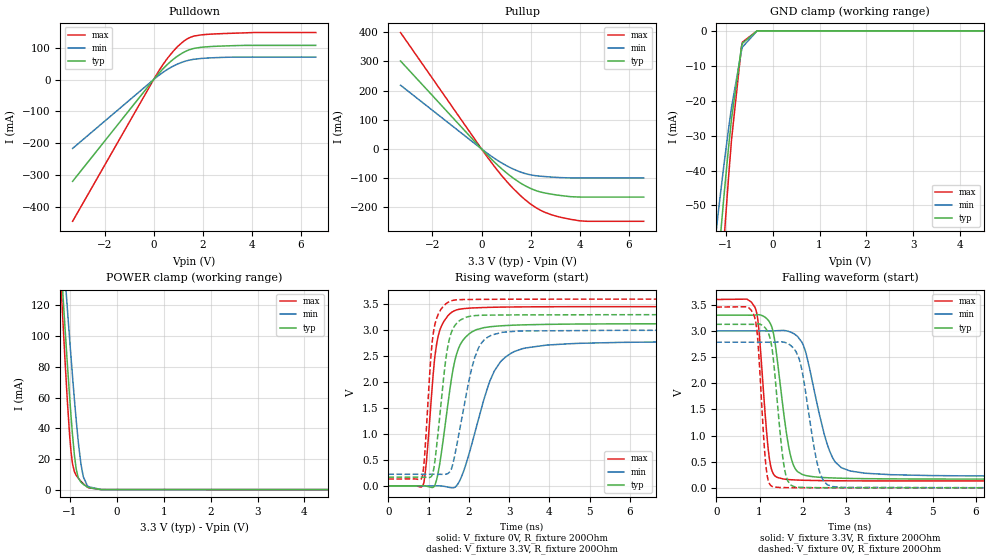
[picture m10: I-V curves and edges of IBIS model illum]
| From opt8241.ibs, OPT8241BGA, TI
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|   illum Model
[Model]   illum
Model_type   I/O
Polarity   Non-Inverting
Enable   Active-High
Vinl = 0.99
Vinh = 2.31
Vmeas = 1.65
Vref = 0
Cref = 2pF
Rref = 200
|   typ   min   max
|   (nom PVT)   (fast PVT)   (slow PVT)
C_comp   2.708e-12   2.507e-12   2.914e-12
[Model spec]
|subparameter
Vinl   0.99   0.90   1.08
Vinh   2.31   2.10   2.52
| Where nom  PVT is Nominal Process, 3.3V, 27C
|   Fast PVT is Strong Process,  3.6V, -40C
|   Slow PVT is Weak Process,   3V, 125C
[Voltage Range]   3.3   3   3.6
|Junction Temperature
[Temperature Range]   27   125   -40
[Pullup Reference]   3.3   3   3.6
[Pulldown Reference]   0   0   0
[Power Clamp Reference]   3.3   3   3.6
[GND Clamp Reference]   0   0   0
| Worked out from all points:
|   slope of the pulldown table from 0 to 0.495 V, typ, clamps not added: 11.6 ohm
|   slope of the pullup table from 0 to 0.495 V, typ, clamps not added: 11.6 ohm
|   falling waveform, V_fixture 3.3V, R_fixture 200Ohm: 20-80 % time 297ps typ, 477ps min, 193ps max; typ from 3.3 V to 0.167 V
|   rising waveform, V_fixture 0V, R_fixture 200Ohm: 20-80 % time 365ps typ, 661ps min, 236ps max; typ from 0 V to 3.13 V
|   rising waveform, V_fixture 3.3V, R_fixture 200Ohm: 20-80 % time 271ps typ, 436ps min, 189ps max; typ from 0.168 V to 3.3 V
|   falling waveform, V_fixture 0V, R_fixture 200Ohm: 20-80 % time 217ps typ, 327ps min, 154ps max; typ from 3.12 V to 0 V
[Pulldown]
|   Voltage   I(typ)   I(min)   I(max)
-3.3V     -319.9mA   -216.5mA   -445.5mA
189mV     17.58mA    11.85mA    24.51mA
462mV     40.27mA    27mA       56.22mA
775.2mV   62.22mA    41.4mA     87.06mA
1.056V    78.05mA    51.51mA    109.5mA
1.251V    86.82mA    56.93mA    122mA
1.596V    97.13mA    63.25mA    135.8mA
2.165V    103mA      67.59mA    142mA
4.032V    107.5mA    70.78mA    147.8mA
6.6V      107.5mA    70.78mA    147.8mA
[GND Clamp]
|   Voltage   I(typ)   I(min)   I(max)
-3.3V     -1.553A    -1.315A    -1.789A
-1.214V   -75.2mA    -58.77mA   -96.04mA
-1.133V   -62.06mA   -49.14mA   -79.22mA
-1.033V   -46.78mA   -37.93mA   -59.46mA
-940.5mV  -33.68mA   -28.26mA   -42.33mA
-876mV    -25.29mA   -22mA      -31.29mA
-663mV    -4.673mA   -5.695mA   -4.527mA
-643.2mV  -3.575mA   -4.674mA   -3.252mA
-330mV    -4.518uA   -17.28uA   -5.664uA
6.6V      0A         0A         0A
[Pullup]
|   Voltage   I(typ)   I(min)   I(max)
-3.3V     301mA      218.2mA    398.3mA
1.2mV     -109.4uA   -79.25uA   -144.7uA
459mV     -39.81mA   -28.44mA   -53.04mA
855mV     -70.54mA   -49.65mA   -94.7mA
1.251V    -97.42mA   -67.29mA   -132mA
1.899V    -131.4mA   -86.9mA    -182.2mA
2.237V    -143.2mA   -91.82mA   -202mA
2.565V    -150.5mA   -94.39mA   -216.4mA
3.032V    -157.2mA   -97.16mA   -229.8mA
3.633V    -163.4mA   -99.07mA   -241mA
4.3V      -164.7mA   -99.07mA   -247.6mA
6.6V      -164.7mA   -99.07mA   -247.6mA
[POWER Clamp]
|   Voltage   I(typ)   I(min)   I(max)
-3.3V     1.269A     1.142A     1.492A
-1.219V   162.5mA    188.8mA    152mA
-1.14V    123.4mA    154.7mA    105.4mA
-1.099V   103.6mA    137.2mA    82.23mA
-1.065V   87.65mA    123mA      64.08mA
-974.4mV  47.89mA    86.2mA     24.75mA
-942mV    35.41mA    73.59mA    16.71mA
-864.6mV  13.5mA     45.43mA    9.371mA
-762mV    4.836mA    16.42mA    5.377mA
-714mV    3.486mA    8.521mA    3.853mA
-600mV    1.284mA    1.875mA    1.166mA
6.6V      0A         0A         0A
[Ramp]
R_load = 200
|   typ   min   max
dV/dt_r   1.87524/3.65085e-10   1.66989/6.58259e-10   2.07288/2.34928e-10
dV/dt_f   1.87941/2.96485e-10   1.66601/4.73757e-10   2.08068/1.93019e-10
[Falling Waveform]
V_fixture = 3.3V
V_fixture_min = 3V
V_fixture_max = 3.6V
R_fixture = 200Ohm
|   Time   V(typ)   V(min)   V(max)
0s        3.3V       3V         3.6V
910ps     3.303V     3V         3.415V
1.22ns    3.181V     2.999V     603.3mV
1.41ns    2.441V     3.004V     199.2mV
1.64ns    944.7mV    2.997V     160.9mV
1.8ns     402.7mV    2.942V     152mV
2.06ns    237.4mV    2.61V      144.2mV
2.56ns    193.7mV    842mV      137.1mV
2.89ns    184.2mV    385mV      134.9mV
8.74ns    167.4mV    223mV      132mV
[Rising Waveform]
V_fixture = 0V
V_fixture_min = 0V
V_fixture_max = 0V
R_fixture = 200Ohm
|   Time   V(typ)   V(min)   V(max)
0s        1.696nV    81.99nV    869pV
870ps     1.132mV    -6.69uV    31.76mV
940ps     -5.176mV   -26.16uV   428.9mV
1.11ns    -28.64mV   335.3uV    2.128V
1.2ns     123.2mV    1.171mV    2.743V
1.64ns    2.376V     -31.75mV   3.376V
1.91ns    2.861V     378.2mV    3.42V
2.52ns    3.067V     2.022V     3.441V
3.14ns    3.099V     2.594V     3.449V
10.73ns   3.126V     2.783V     3.455V
[Rising Waveform]
V_fixture = 3.3V
V_fixture_min = 3V
V_fixture_max = 3.6V
R_fixture = 200Ohm
|   Time   V(typ)   V(min)   V(max)
0s        167.6mV    223.3mV    132mV
840ps     168.5mV    223.3mV    170.7mV
900ps     167.3mV    223.2mV    584.2mV
1.09ns    214.5mV    223.4mV    2.783V
1.24ns    1.068V     223.8mV    3.312V
1.51ns    2.814V     258.8mV    3.55V
1.71ns    3.147V     831.9mV    3.588V
2.14ns    3.282V     2.464V     3.594V
2.56ns    3.292V     2.905V     3.596V
8.95ns    3.3V       3V         3.6V
[Falling Waveform]
V_fixture = 0V
V_fixture_min = 0V
V_fixture_max = 0V
R_fixture = 200Ohm
|   Time   V(typ)   V(min)   V(max)
0s        3.125V     2.783V     3.455V
880ps     3.127V     2.783V     3.278V
960ps     3.133V     2.783V     2.816V
1.14ns    3.048V     2.783V     481.1mV
1.28ns    2.709V     2.783V     31.99mV
1.56ns    446.4mV    2.784V     5.518mV
1.78ns    27.94mV    2.674V     3.748mV
2.36ns    3.933mV    377.8mV    1.443mV
2.57ns    2.99mV     57.07mV    1.164mV
8.21ns    -40.21uV   35.42uV    -4.109uV
